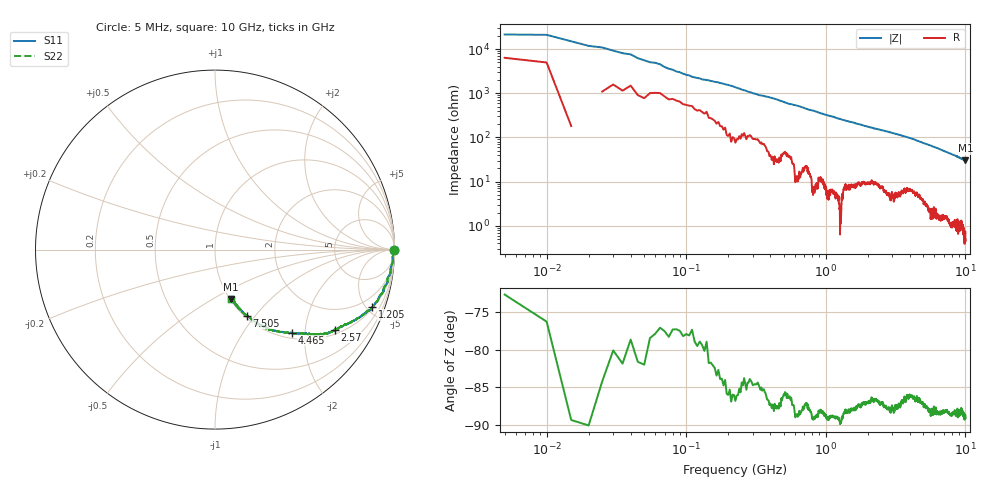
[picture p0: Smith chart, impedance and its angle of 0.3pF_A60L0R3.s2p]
! Amotech Co.,Ltd.
! http://www.amotech.co.kr/
! Part Number: A60L0R3
! These Parameters are Measured in Series Mode Connection
! Operation Temp=25[degC], DC Bias Voltage=0[V]
! Freq. Start=5[MHz] Stop=10[GHz], 2000[Steps]
! Date: Monday, July 14, 2020, 09:24:43
# GHZ S RI R 50.000000
!Freq.(Hz) S11(Real) S11(Imag) S21(Real) S21(Imag) S12(Real) S12(Imag) S22(Real) S22(Imag)
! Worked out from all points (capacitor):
!   2000 points, 5 MHz to 10 GHz, reference 50 ohm
!   read as one part in series: C = 606 fF near 55 MHz
!   lowest |Z| = 30.2 ohm at 10 GHz (marker M1)
!   S11 on the Smith chart (normalised r, x): 5 MHz: open; 1.205 GHz: 1.10, -5.45; 2.57 GHz: 1.15, -2.88; 4.465 GHz: 1.11, -1.71; 7.505 GHz: 1.03, -0.90; 10 GHz: 1.01, -0.60
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0.005  0.9986 -0.00447  0.00141 0.00447  0.00141 0.00447  0.9986 -0.00447
0.03  0.998 -0.0107  0.00198 0.0107  0.00198 0.0107  0.998 -0.0107
0.075  0.9936 -0.0271  0.00637 0.0271  0.00637 0.0271  0.9936 -0.0271
0.095  0.9914 -0.0349  0.00856 0.0349  0.00856 0.0349  0.9914 -0.0349
0.115  0.9898 -0.0423  0.0102 0.0423  0.0102 0.0423  0.9898 -0.0423
0.16  0.9898 -0.054  0.0102 0.054  0.0102 0.054  0.9898 -0.054
0.295  0.9813 -0.0948  0.0187 0.0948  0.0187 0.0948  0.9813 -0.0948
0.35  0.9788 -0.1095  0.0212 0.1095  0.0212 0.1095  0.9788 -0.1095
0.51  0.9632 -0.1537  0.0368 0.1537  0.0368 0.1537  0.9632 -0.1537
0.715  0.9441 -0.2065  0.0559 0.2065  0.0559 0.2065  0.9441 -0.2065
0.945  0.9156 -0.2634  0.0844 0.2634  0.0844 0.2634  0.9156 -0.2634
1.205  0.8767 -0.3195  0.1233 0.3195  0.1233 0.3195  0.8767 -0.3195
1.675  0.796 -0.3826  0.204 0.3826  0.204 0.3826  0.796 -0.3826
2.57  0.6665 -0.4462  0.3335 0.4462  0.3335 0.4462  0.6665 -0.4462
3.34  0.5652 -0.4718  0.4348 0.4718  0.4348 0.4718  0.5652 -0.4718
4.465  0.4283 -0.463  0.5717 0.463  0.5717 0.463  0.4283 -0.463
5.005  0.3642 -0.4588  0.6358 0.4588  0.6358 0.4588  0.3642 -0.4588
5.805  0.2842 -0.438  0.7158 0.438  0.7158 0.438  0.2842 -0.438
6.67  0.2252 -0.4046  0.7748 0.4046  0.7748 0.4046  0.2252 -0.4046
7.505  0.1768 -0.3673  0.8232 0.3673  0.8232 0.3673  0.1768 -0.3673
8.335  0.1413 -0.3356  0.8587 0.3356  0.8587 0.3356  0.1413 -0.3356
10  0.0876 -0.2746  0.9124 0.2746  0.9124 0.2746  0.0876 -0.2746
